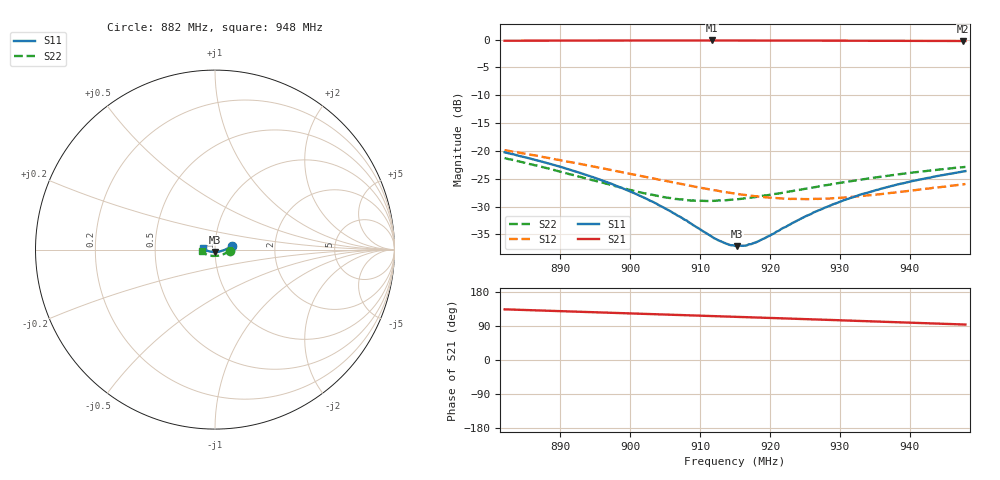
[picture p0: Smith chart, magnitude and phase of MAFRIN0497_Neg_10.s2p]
!Part Number:  MAFRIN0497
!Name:  MariaCraven
!Comments:  1
!Thu 30/Sep/2004  3:12:36 PM
!Temperature:  -10
# MHZ  S  DB  R  50
!Freq  S11(dB)  S11(ang)  S21(dB)  S21(ang)  S12(dB)  S12(ang)  S22(dB)  S22(ang)
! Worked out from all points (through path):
!   201 points, 882 MHz to 948 MHz, reference 50 ohm
!   highest |S21| = -0.17 dB at 911.7 MHz (marker M1); lowest = -0.3 dB at 947.7 MHz (marker M2)
!   lowest |S11| = -37.1 dB at 915.3 MHz (marker M3), VSWR 1.03, Z = 50.1 - j1.4 ohm
!   |S11| at or under -10 dB: start of sweep to end of sweep
!   |S22| runs from -29.0 to -21.3 dB; largest |S21 - S12| = 0.97
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882  -20.25 12.8  -0.22 133.7  -19.87 105.5  -21.27 -3.6
888.6  -22.35 7.0  -0.20 129.8  -21.34 105.5  -23.28 -14.4
893.22  -24.13 2.0  -0.19 127.1  -22.43 106.8  -24.79 -23.9
898.83  -26.68 -5.4  -0.18 123.8  -23.81 109.5  -26.64 -39.3
902.46  -28.68 -12.3  -0.18 121.6  -24.72 112.1  -27.71 -51.5
904.11  -29.76 -16.3  -0.18 120.7  -25.17 113.7  -28.14 -58.0
907.74  -32.33 -28.1  -0.18 118.5  -26.07 118.0  -28.81 -73.0
911.7  -35.42 -51.4  -0.17 116.1  -26.97 123.8  -28.98 -90.3
913.68  -36.62 -69.1  -0.18 114.9  -27.42 127.2  -28.86 -98.4
915  -37.04 -83.2  -0.18 114.1  -27.65 129.8  -28.73 -103.5
915.33  -37.10 -86.5  -0.18 113.9  -27.70 130.6  -28.68 -104.8
916.65  -36.99 -100.9  -0.19 113.1  -27.94 133.1  -28.50 -109.6
918.3  -36.26 -116.2  -0.19 112.0  -28.20 136.6  -28.18 -115.3
920.61  -34.82 -133.1  -0.19 110.6  -28.43 141.8  -27.73 -122.7
922.92  -33.19 -144.6  -0.20 109.2  -28.63 147.0  -27.25 -129.1
926.22  -31.07 -155.7  -0.20 107.2  -28.63 154.6  -26.56 -137.1
929.19  -29.52 -162.9  -0.21 105.4  -28.49 160.8  -25.92 -143.6
933.15  -27.76 -169.9  -0.22 102.8  -28.10 168.2  -25.14 -150.8
937.11  -26.41 -175.4  -0.23 100.4  -27.58 174.3  -24.43 -157.2
940.41  -25.41 -179.6  -0.24 98.3  -27.10 178.4  -23.89 -162.0
947.67  -23.70 172.4  -0.27 93.7  -26.01 -175.0  -22.92 -171.7
948  -23.63 172.1  -0.27 93.5  -25.94 -174.8  -22.87 -172.0
